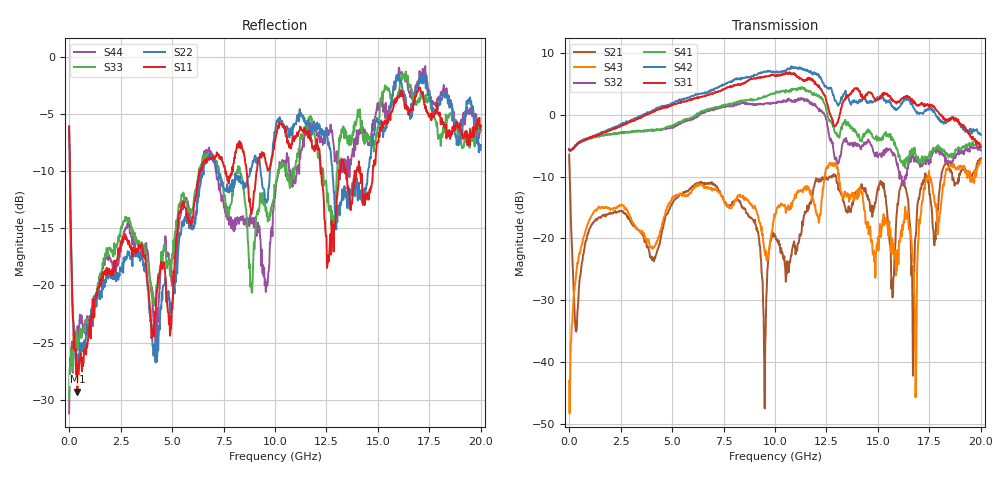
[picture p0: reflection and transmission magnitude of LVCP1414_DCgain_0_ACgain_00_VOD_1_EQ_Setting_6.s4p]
!Agilent Technologies,N5230A,MY46400459,A.07.50.48
!Agilent N5230A: A.07.50.48
!Date: Tuesday, April 17, 2012 18:27:44
!Correction: S11(Full 4 Port(1,2,3,4))
!S12(Full 4 Port(1,2,3,4))
!S13(Full 4 Port(1,2,3,4))
!S14(Full 4 Port(1,2,3,4))
!S21(Full 4 Port(1,2,3,4))
!S22(Full 4 Port(1,2,3,4))
!S23(Full 4 Port(1,2,3,4))
!S24(Full 4 Port(1,2,3,4))
!S31(Full 4 Port(1,2,3,4))
!S32(Full 4 Port(1,2,3,4))
!S33(Full 4 Port(1,2,3,4))
!S34(Full 4 Port(1,2,3,4))
!S41(Full 4 Port(1,2,3,4))
!S42(Full 4 Port(1,2,3,4))
!S43(Full 4 Port(1,2,3,4))
!S44(Full 4 Port(1,2,3,4))
!S4P File: Measurements: <S11,S12,S13,S14>,
!<S21,S22,S23,S24>,
!<S31,S32,S33,S34>,
!<S41,S42,S43,S44>:
# Hz S  dB  R 50
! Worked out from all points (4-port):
!   801 points, 300 kHz to 20 GHz, reference 50 ohm
!   strongest paths, dB at 300 kHz, 5 GHz, 10 GHz, 15 GHz, 20 GHz:
!     S31: -5.6, 1.5, 6.2, 2.4, -5.2
!     S42: -5.7, 1.9, 6.8, 2.7, -3.3
!     S41: -5.6, -1.8, 3.3, -3.7, -4.9
!     S32: -5.6, -2.1, 1.8, -6.9, -5.8
!     S43: -43.0, -13.4, -16.5, -19.8, -7.3
!     S21: -6.5, -14.4, -19.7, -11.7, -7.1
!   lowest |S11| = -29.3 dB at 400.3 MHz (marker M1), VSWR 1.07, Z = 53.2 + j1.44 ohm
!   |S11| at or under -10 dB: 37.57 MHz to 6.324 GHz (6.286 GHz wide, 198 % of centre); 12.25 GHz to 13.12 GHz (866.2 MHz wide, 6.83 % of centre); 14.14 GHz to 14.75 GHz (609.8 MHz wide, 4.22 % of centre)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
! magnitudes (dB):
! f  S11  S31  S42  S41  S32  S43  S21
! 300 kHz  -6.1  -5.6  -5.7  -5.6  -5.6  -43.0  -6.5
! 400.3 MHz  -29.3  -4.7  -4.7  -4.8  -4.8  -23.9  -32.0
! 10 GHz  -7.4  6.2  6.8  3.3  1.8  -16.5  -19.7
! 12.88 GHz  -14.7  -1.8  2.7  -2.5  -6.4  -8.0  -9.8
! 16.8 GHz  -3.4  1.9  0.8  -6.3  -7.0  -32.3  -20.3
! 17.38 GHz  -4.7  1.5  0.7  -6.8  -7.3  -10.7  -10.1
! 20 GHz  -6.0  -5.2  -3.3  -4.9  -5.8  -7.3  -7.1
